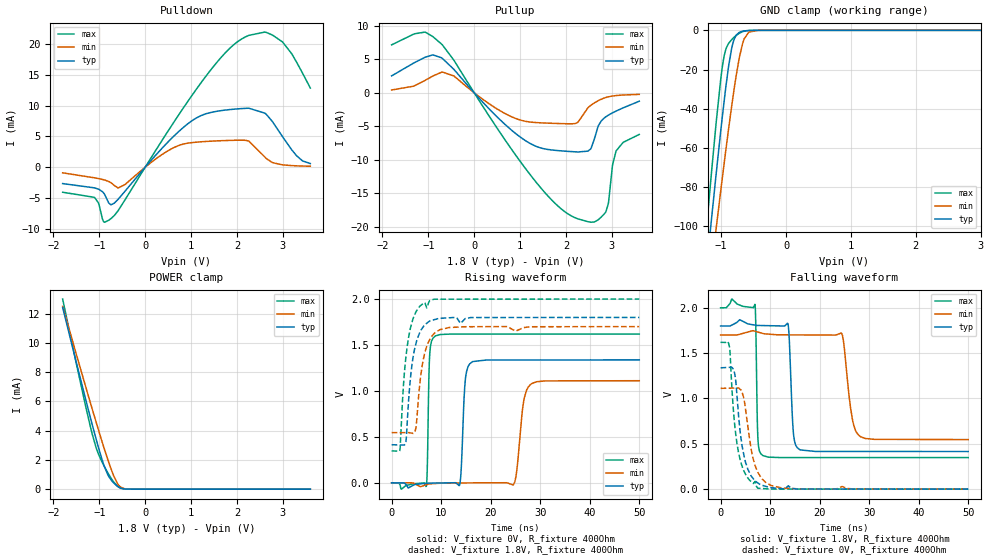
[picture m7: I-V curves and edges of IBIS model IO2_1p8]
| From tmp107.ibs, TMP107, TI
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|   Model
[Model]   IO2_1p8
Model_type   I/O
Polarity   Non-Inverting
Enable   Active-Low
Vinl = 0.54
Vinh = 1.26
Vmeas = 0.9
Vref = 0
Cref = 1pF
Rref = 100000
|   typ   min   max
C_comp   1.060pF   1.035pF   1.082pF
[Voltage Range]   1.8   1.7   2
[Temperature Range]   25   125   -55
[Pullup Reference]   1.8   1.7   2
[Pulldown Reference]   0   0   -0
[Power Clamp Reference]   1.8   1.7   2
[GND Clamp Reference]   0   0   0
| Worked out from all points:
|   slope of the pulldown table from 0 to 0.27 V, typ, clamps not added: 118 ohm
|   slope of the pullup table from 0 to 0.27 V, typ, clamps not added: 135 ohm
|   GND clamp passes 1 mA (typ) near -0.72 V on its own axis
|   POWER clamp passes 1 mA (typ) near -0.82 V on its own axis
|   falling waveform, V_fixture 1.8V, R_fixture 400Ohm: 20-80 % time 633ps typ, 1.45ns min, 299ps max; typ from 1.8 V to 0.415 V
|   rising waveform, V_fixture 0V, R_fixture 400Ohm: 20-80 % time 647ps typ, 1.22ns min, 339ps max; typ from 0 V to 1.34 V
|   rising waveform, V_fixture 1.8V, R_fixture 400Ohm: 20-80 % time 1.76ns typ, 1.79ns min, 1.74ns max; typ from 0.415 V to 1.8 V
|   falling waveform, V_fixture 0V, R_fixture 400Ohm: 20-80 % time 1.96ns typ, 2.21ns min, 1.84ns max; typ from 1.34 V to 0 V
[Pulldown]
|   Voltage   I(typ)   I(min)   I(max)
-1.8V     -2.666mA   -916.2uA   -4.076mA
-1.109V   -3.362mA   -1.726mA   -4.902mA
-909mV    -4.177mA   -2.037mA   -8.834mA
-747mV    -6.118mA   -2.522mA   -8.368mA
-444.6mV  -3.943mA   -2.846mA   -5.362mA
462.6mV   3.837mA    2.519mA    5.47mA
997.2mV   7.442mA    3.982mA    11.44mA
1.748V    9.298mA    4.335mA    18.63mA
2.255V    9.593mA    4.243mA    21.44mA
2.639V    8.605mA    1.43mA     21.93mA
2.995V    4.955mA    375.9uA    20.37mA
3.6V      590.1uA    156.3uA    12.89mA
[GND Clamp]
|   Voltage   I(typ)   I(min)   I(max)
-1.8V     -318.4mA   -308.8mA   -326.7mA
-1.222V   -120.5mA   -141.6mA   -99.69mA
-1.152V   -97.35mA   -121.9mA   -73.59mA
-1.076V   -73.02mA   -100.9mA   -46.83mA
-1.006V   -51.29mA   -81.81mA   -24.84mA
-952.2mV  -35.56mA   -67.45mA   -12.75mA
-887.4mV  -18.85mA   -50.79mA   -6.767mA
-833.4mV  -8.469mA   -37.6mA    -4.592mA
-720mV    -1.046mA   -13.92mA   -1.493mA
-644.4mV  -285.9uA   -4.287mA   -441.6uA
-444.6mV  -3.48uA    -39.44uA   -2.446uA
3.6V      0A         0A         0A
[Pullup]
|   Voltage   I(typ)   I(min)   I(max)
-1.8V     2.51mA     410.1uA    7.13mA
-1.071V   5.28mA     1.835mA    9.033mA
-714.6mV  5.211mA    3.045mA    7.269mA
1.067V    -6.904mA   -4.18mA    -10.82mA
1.748V    -8.566mA   -4.564mA   -16.37mA
2.266V    -8.822mA   -4.366mA   -18.79mA
2.542V    -8.367mA   -1.877mA   -19.28mA
2.86V     -3.636mA   -730uA     -17.85mA
2.925V    -3.342mA   -607.7uA   -16.53mA
3.017V    -2.993mA   -489.3uA   -10.76mA
3.092V    -2.738mA   -423.6uA   -8.715mA
3.6V      -1.26mA    -243.5uA   -6.206mA
[POWER Clamp]
|   Voltage   I(typ)   I(min)   I(max)
-1.8V     12.41mA    12.49mA    12.99mA
-1.298V   6.128mA    6.997mA    5.65mA
-1.163V   4.498mA    5.551mA    3.857mA
-1.071V   3.426mA    4.583mA    2.841mA
-1.022V   2.879mA    4.078mA    2.424mA
-919.8mV  1.814mA    3.032mA    1.724mA
-811.8mV  961.8uA    1.983mA    1.093mA
-693mV    440.4uA    956.5uA    513.3uA
-579.6mV  145.7uA    277.2uA    137.6uA
-444.6mV  12.77uA    26.7uA     6.023uA
-342mV    881.2nA    3.008uA    185nA
3.6V      0A         0A         0A
[Ramp]
R_load = 400
|   typ   min   max
dV/dt_r   0.80269/6.38754e-10   0.666748/1.2169e-09   0.971371/3.38012e-10
dV/dt_f   0.83113/6.31413e-10   0.692088/1.45049e-09   0.991465/2.98509e-10
[Falling Waveform]
V_fixture = 1.8V
V_fixture_min = 1.7V
V_fixture_max = 2V
R_fixture = 400Ohm
C_fixture = 0F
|   Time   V(typ)   V(min)   V(max)
0s        1.8V       1.7V       2V
6.94ns    1.809V     1.742V     2.038V
7.53ns    1.805V     1.733V     563.1mV
8.529ns   1.804V     1.717V     370.3mV
13.62ns   1.82V      1.702V     348.1mV
14.71ns   619.3mV    1.701V     348.1mV
15.99ns   435mV      1.701V     348mV
24.43ns   415.4mV    1.719V     347.9mV
28.29ns   415.3mV    577.3mV    347.9mV
50ns      414.8mV    546.5mV    347.6mV
[Rising Waveform]
V_fixture = 0V
V_fixture_min = 0V
V_fixture_max = 0V
R_fixture = 400Ohm
C_fixture = 0F
|   Time   V(typ)   V(min)   V(max)
0s        96.49nV    242.3nV    109.3nV
7.013ns   -4.438mV   -20.91mV   -36.64mV
7.686ns   -3.528mV   -10.96mV   1.392V
8.827ns   -2.537mV   -7.489mV   1.598V
13.71ns   -26.47mV   -1.162mV   1.619V
14.88ns   1.121V     -900.2uV   1.619V
16.3ns    1.318V     -585.3uV   1.619V
24.6ns    1.337V     -20.53mV   1.619V
28.29ns   1.337V     1.08V      1.619V
50ns      1.338V     1.111V     1.619V
[Rising Waveform]
V_fixture = 1.8V
V_fixture_min = 1.7V
V_fixture_max = 2V
R_fixture = 400Ohm
C_fixture = 0F
|   Time   V(typ)   V(min)   V(max)
0s        414.8mV    546.5mV    347.6mV
1.714ns   412.2mV    546.6mV    370.4mV
2.216ns   411.5mV    546.6mV    910.9mV
2.774ns   421.5mV    546.7mV    1.31V
3.766ns   1.121V     543.8mV    1.677V
4.711ns   1.473V     554.1mV    1.836V
6.569ns   1.713V     1.387V     1.961V
8.705ns   1.777V     1.632V     1.999V
11.6ns    1.796V     1.69V      1.999V
50ns      1.8V       1.7V       2V
[Falling Waveform]
|Gnd
V_fixture = 0V
V_fixture_min = 0V
V_fixture_max = 0V
R_fixture = 400Ohm
C_fixture = 0F
|   Time   V(typ)   V(min)   V(max)
0s        1.338V     1.111V     1.619V
1.792ns   1.343V     1.114V     1.57V
2.851ns   1.272V     1.115V     707.3mV
3.638ns   807.4mV    1.116V     399.2mV
4.277ns   502.4mV    1.079V     264mV
5.499ns   219.6mV    694.7mV    123mV
6.534ns   119.5mV    344.3mV    65.57mV
7.507ns   68.75mV    187.7mV    10.09mV
12.41ns   4.798mV    12.59mV    190.2uV
50ns      370.4nV    612.1nV    256.4nV
